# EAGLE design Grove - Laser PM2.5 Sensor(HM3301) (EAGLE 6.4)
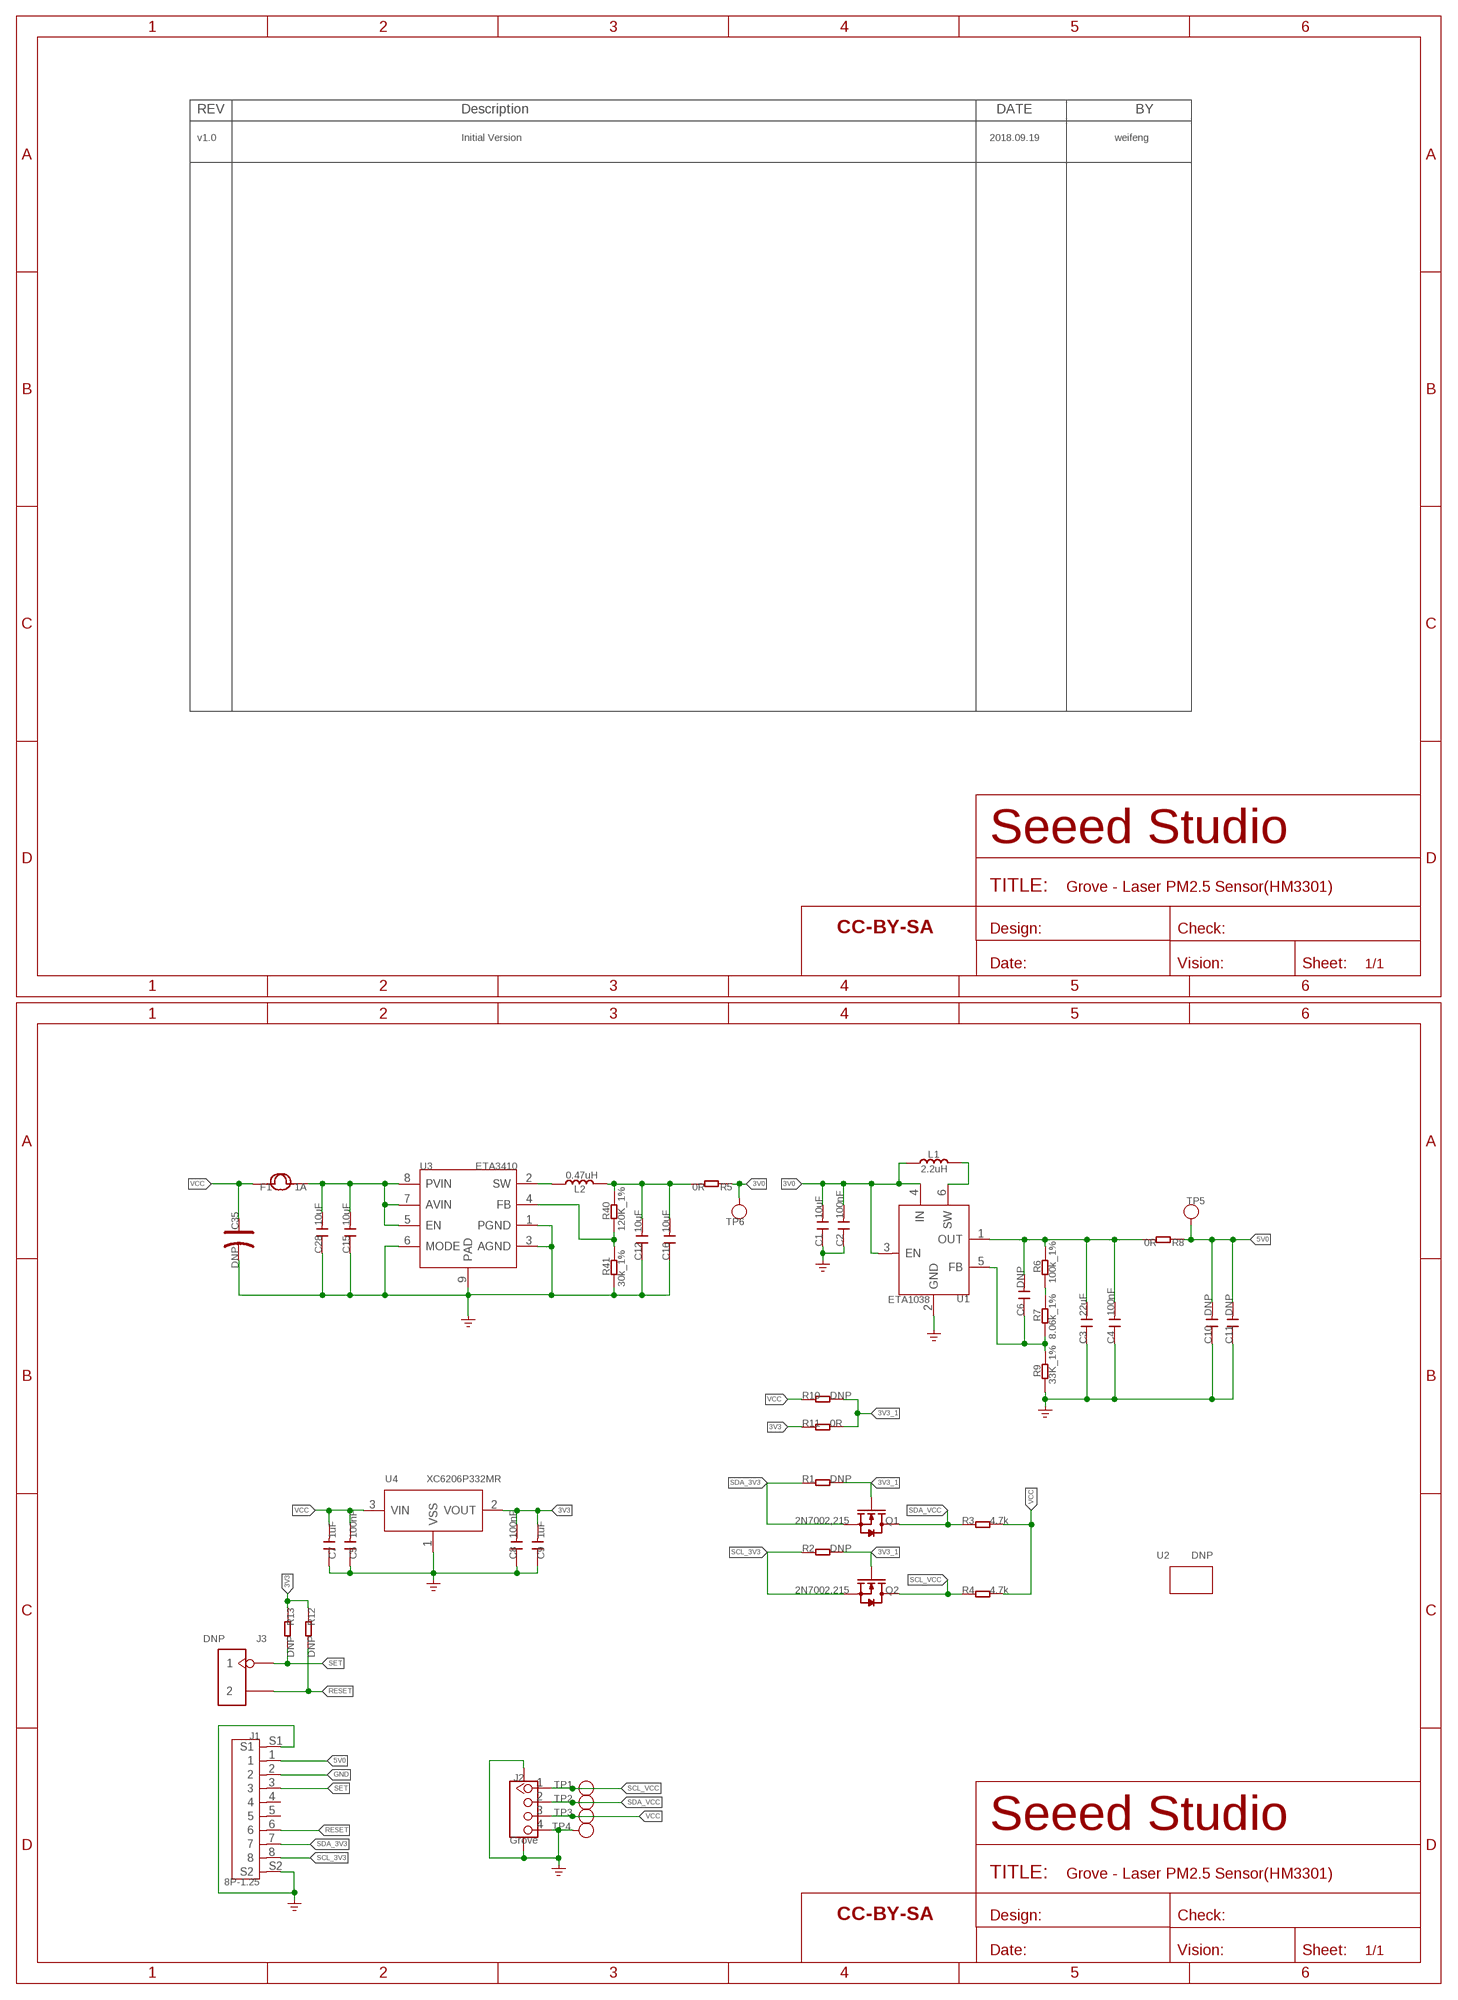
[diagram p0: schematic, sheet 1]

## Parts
C1  10uF  C-0603  [C0603]
C2  100nF  C-0603  [C0603]
C3  22uF  C-0805  [C0805]
C4  100nF  C-0603  [C0603]
C5  100nF  C-0603  [C0603]
C6  DNP  C-0603  [C0603]
C7  1uF  C-0603  [C0603]
C8  100nF  C-0603  [C0603]
C9  1uF  C-0603  [C0603]
C10  DNP  C-0805  [C0805]
C11  DNP  C-0603  [C0603]
C12  10uF  C-0603  [C0603]
C15  10uF  C-0603  [C0603]
C16  10uF  C-0603  [C0603]
C28  10uF  C-0603  [C0603]
C35  DNP  CAP-POLAR-AVX-B  [AVX-B]
F1  1A  FUSE-0805  [F0805]
FR1  SEEEDSTUDIO-OPEN-SCH-FRAME  [SEEEDSTUDIO-PCB-FRAME]
J1  8P-1.25  HEADER-8+2P  [HEADER8+2P-SMD-1.25-15X3.5MM]
J2  Grove  GROVE-CONNECTOR-SMD'90D'  [HW4-SMD-2.0-90D]
J3  DNP  HEADER-2P-65/35MIL  [H2-2.54]
L1  2.2uH  INDUCTOR/FERRITE-BEAD'0806'  [L0806]
L2  0.47uH  L-MPM201610SR33_T  [L201610]
Q1  2N7002,215  MOSFET-N'SOT23'  [SOT-23]
Q2  2N7002,215  MOSFET-N'SOT23'  [SOT-23]
R1  DNP  R-0603  [R0603]
R2  DNP  R-0603  [R0603]
R3  4.7k  R-0603  [R0603]
R4  4.7k  R-0603  [R0603]
R5  0R  R-0603  [R0603]
R6  100k_1%  R-0603  [R0603]
R7  8.06k_1%  R-0603  [R0603]
R8  0R  R-0603  [R0603]
R9  33K_1%  R-0603  [R0603]
R10  DNP  R-0603  [R0603]
R11  0R  R-0603  [R0603]
R12  DNP  R-0603  [R0603]
R13  DNP  R-0603  [R0603]
R40  120K_1%  R-0603  [R0603]
R41  30k_1%  R-0603  [R0603]
TP1  TEST-POINT'4545'  [TP-D45MIL]
TP2  TEST-POINT'4545'  [TP-D45MIL]
TP3  TEST-POINT'4545'  [TP-D45MIL]
TP4  TEST-POINT'4545'  [TP-D45MIL]
TP5  TEST-POINT'4545'  [TP-D45MIL]
TP6  TEST-POINT'4545'  [TP-D45MIL]
U1  ETA1038  CONVERTER-ETA1038  [SOT-23-6]
U2  DNP  GROVE-80X40MM  [GROVE-80X40MM]
U3  ETA3410  CONVERTER-ETA3410  [DFN8G-0.5-2X2MM]
U4  XC6206P332MR  PMIC-XC6206PMR  [SOT-23]
U$4  SEEEDSTUDIO-OPEN-SCH-FRAME  [SEEEDSTUDIO-PCB-FRAME]

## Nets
3V0: C1.2 C2.2 L1.1 R5.1 TP6.T U1.3(EN) U1.4(IN)
3V3: C8.2 C9.2 R11.1 R12.1 R13.1 U4.2(VOUT)
3V3_1: Q1.1(G) Q2.1(G) R1.2 R2.2 R10.2 R11.2
5V0: C10.2 C11.2 J1.1 R8.1 TP5.T
GND: C1.1 C2.1 C3.1 C4.1 C5.1 C7.1 C8.1 C9.1 C10.1 C11.1 C12.1 C15.1 C16.1 C28.1 C35.- J1.2 J1.S1 J1.S2 J2.4 J2.SS1 J2.SS2 R9.2 R41.1 TP4.T U1.2(GND) U3.1(PGND) U3.3(AGND) U3.6(MODE) U3.9(PAD) U4.1(VSS) ; supply symbol labelled GND_POWER
N$7: C15.2 C28.2 F1.2 U3.5(EN) U3.7(AVIN) U3.8(PVIN)
N$8: L1.2 U1.6(SW)
N$9: C3.2 C4.2 C6.2 R6.1 R8.2 U1.1(OUT)
N$10: R6.2 R7.1
N$11: C6.1 R7.2 R9.1 U1.5(FB)
N$21: R40.1 R41.2 U3.4(FB)
N$29: L2.1 U3.2(SW)
N$64: C12.2 C16.2 L2.2 R5.2 R40.2
RESET: J1.6 J3.2 R12.2
SCL_3V3: J1.8 Q2.2(S) R2.1
SCL_VCC: J2.1 Q2.3(D) R4.1 TP1.T
SDA_3V3: J1.7 Q1.2(S) R1.1
SDA_VCC: J2.2 Q1.3(D) R3.1 TP2.T
SET: J1.3 J3.1 R13.2
VCC: C5.2 C7.2 C35.+ F1.1 J2.3 R3.2 R4.2 R10.1 TP3.T U4.3(VIN)
Unconnected: J1.4 J1.5

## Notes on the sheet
- v1.0 | Initial Version | 2018.09.19 | weifeng
- Vout=(R3+R4+R9)/R9x1.17V

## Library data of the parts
C1-C12 C15 C16 C28 = Discrete-small:C*: Ceramic Capacitors
C35 = Discrete-new:CAP-POLAR: Electrolytic Capacitors,Tantalum Capacitors and Super Capacitors
F1 = Discrete-new:FUSE
FR1 U$4 = moudle-new:SEEEDSTUDIO-OPEN-SCH-FRAME
J1 = Connector-new:HEADER-8+2P
J2 = Connector-new:GROVE-CONNECTOR-SMD: 4P-SMD-2.0:320110030;4P-SMD-2.0-90D:320110032
J3 = Connector-new:HEADER-2P
L1 = Discrete-new:INDUCTOR/FERRITE-BEAD
L2 = Discrete-new:L
Q1 Q2 = Discrete-new:MOSFET-N
R1-R13 R40 R41 = Discrete-small:R*
TP1-TP6 = Discrete-new:TEST-POINT; PARTNO: DNP
U1 = IC-new:CONVERTER-ETA1038
U2 = moudle-new:GROVE
U3 = IC-new:CONVERTER-ETA3410: 3MHZ 2A High Step-Down Converter in DFN2x2-8L Package
U4 = IC-new:PMIC-XC6206P: LOW ESR Cap.Compatible Positive Voltage Regulators

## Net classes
3 usbvcc: width 0.203 mm, drill 0.305 mm, clearance 0.203 mm

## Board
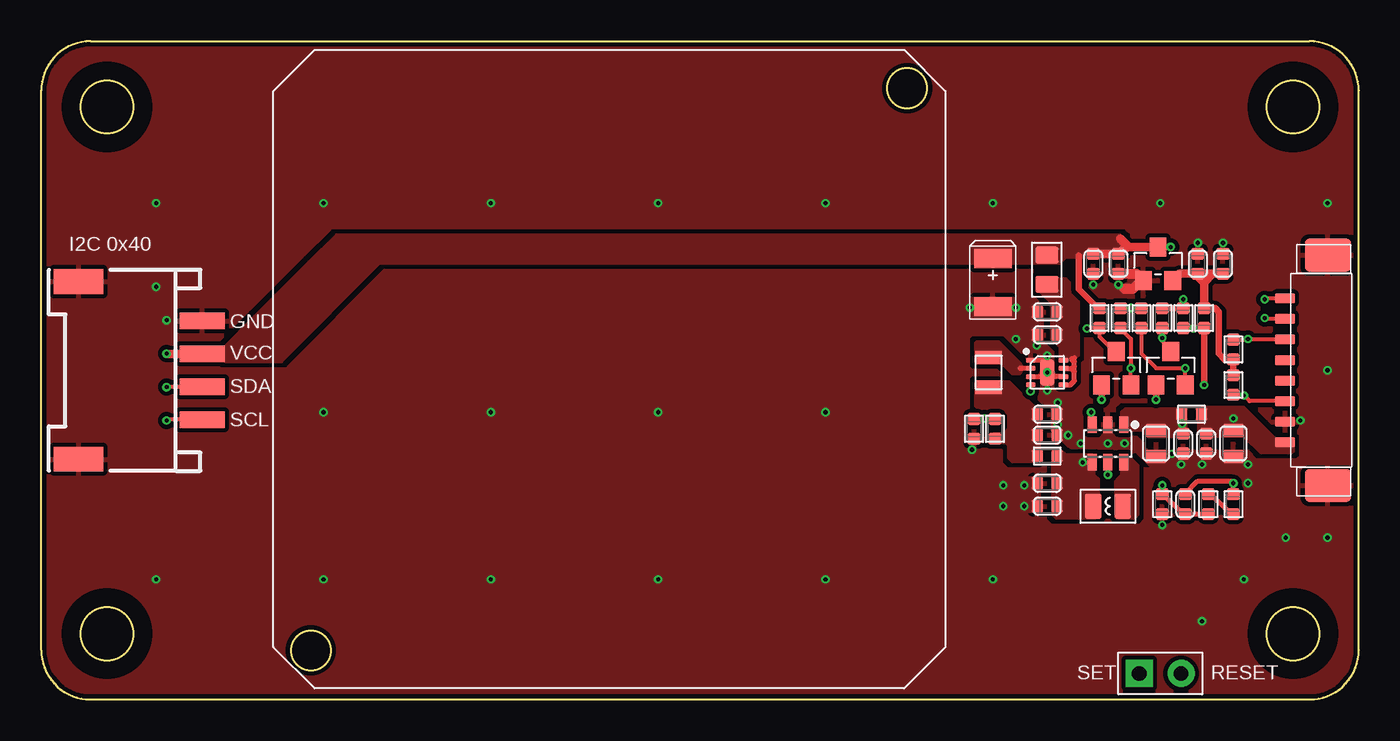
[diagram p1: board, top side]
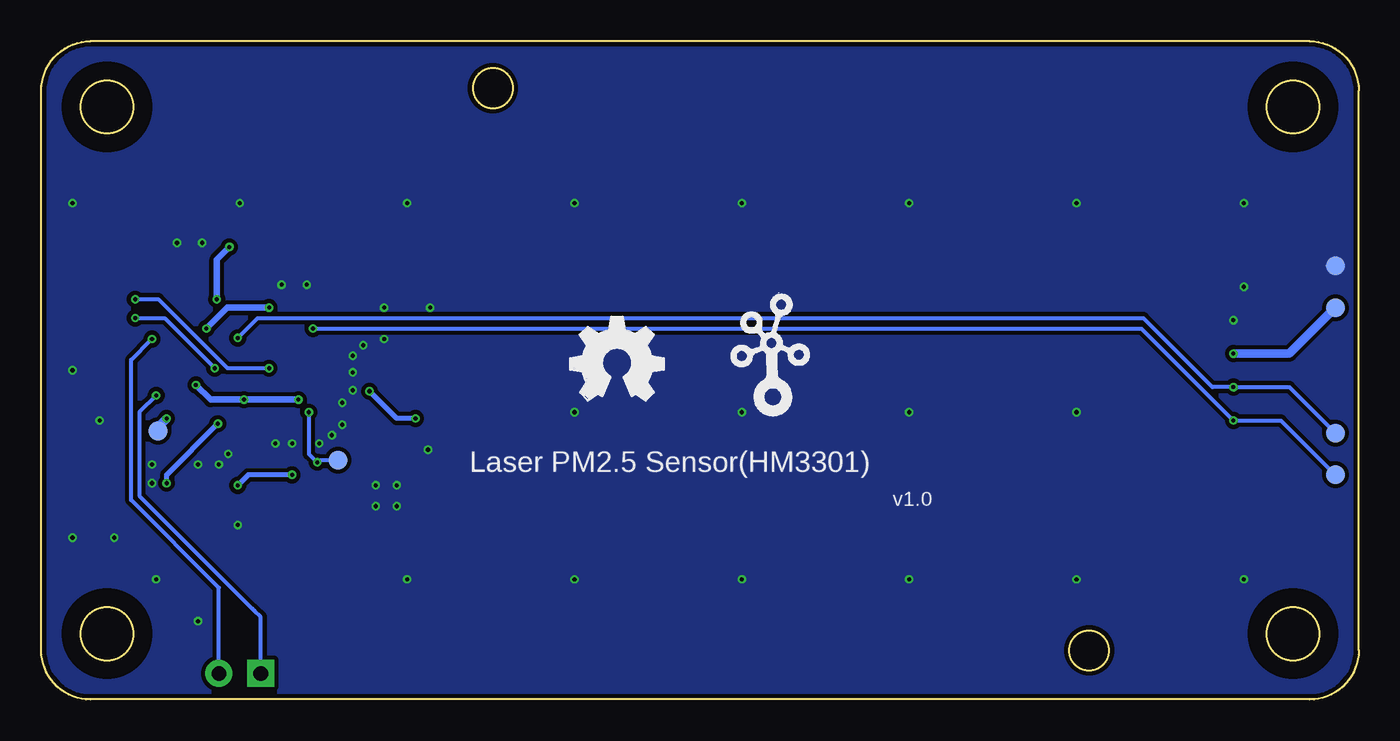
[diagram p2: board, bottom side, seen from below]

Size 80 x 40 mm. Coordinates in mm from the lower left corner, seen from the top.
Outline: circle at 16.38,2.98 radius 1.2
Outline: circle at 52.57,37.14 radius 1.2
Copper layers (1*16): Top 0.035mm / dielectric 1.5mm / Bottom 0.035mm
Design rules "SeeedStudio_2layer_DRU_no_angle_20140221 *": minimum track width 1mil, minimum drill 10mil, track to track 6mil, track to pad 6mil, pad to pad 6mil, via to via 6mil, smd to smd 0mil, copper to edge 10mil, drill to drill 10mil, minimum pad ring 4mil, minimum via ring 4mil, stop-mask expansion 2mil, vias tented up to drill 25mil, thermal gap 10mil

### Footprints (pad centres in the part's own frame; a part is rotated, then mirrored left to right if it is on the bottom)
C0603 = smd 0.762 x 0.696: 1 0,0.602; 2 0,-0.602
C0805 = smd 0.819 x 1.27: 1 -0.79,0; 2 0.79,0
AVX-B = smd 1.143 x 2.286: + 1.46,0; - -1.46,0
F0805 = smd 1.016 x 1.397: 1 -0.889,0; 2 0.889,0
HEADER8+2P-SMD-1.25-15X3.5MM = smd 0.6 x 1.2: 1 -4.375,2.2; 2 -3.125,2.2; 3 -1.875,2.2; 4 -0.625,2.2; 5 0.625,2.2; 6 1.875,2.2; 7 3.125,2.2; 8 4.375,2.2 | smd 2 x 2.8: S1 -7,-0.4; S2 7,-0.4
HW4-SMD-2.0-90D = smd 1.01 x 2.74: 1 -3,-0.1; 2 -1,-0.1; 3 1,-0.1; 4 3,-0.1 | smd 1.5 x 3: SS1 -5.4,7.4; SS2 5.4,7.4
H2-2.54 = drill 0.889 pad 1.651 square: 1 0,1.27 | drill 0.889 pad 1.651: 2 0,-1.27
L0806 = smd 1.016 x 1.524: 1 -0.889,0; 2 0.889,0
L201610 = smd 0.8 x 1.6: 1 -0.9,0; 2 0.9,0
SOT-23 = smd 1.143 x 1.016: 1 1.016,-0.889; 2 1.016,0.889; 3 -1.016,0
R0603 = smd 0.762 x 0.696: 1 0,0.602; 2 0,-0.602
TP-D45MIL = smd 1.143 x 1.143: T 0,0
SOT-23-6 = smd 0.55 x 1.016: 1 -0.95,-1.143; 2 0,-1.143; 3 0.95,-1.143; 4 0.95,1.143; 5 0,1.143; 6 -0.95,1.143
DFN8G-0.5-2X2MM = smd 0.6 x 0.3: 1 -1,0.75; 2 -1,0.25; 3 -1,-0.25; 4 -1,-0.75; 5 1,-0.75; 6 1,-0.25; 7 1,0.25; 8 1,0.75 | smd 0.9 x 1.6: 9 0,0
SOT-23' = smd 1.016 x 1.143: 1 -0.889,-1.016; 2 0.889,-1.016; 3 0,1.016

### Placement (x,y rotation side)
C1  61.08,11.74 90 top
C2  61.08,13.14 90 top
C3  67.69,15.55 90 top
C4  69.34,15.55 180 top
C5  65.4,26.48 180 top
C6  69.46,11.87 180 top
C7  63.88,26.48 180 top
C8  71.75,26.48 0 top
C9  70.23,26.48 0 top
C10  72.38,15.55 90 top
C11  70.73,15.55 180 top
C12  61.08,17.33 270 top
C15  61.08,22.16 90 top
C16  61.08,16.06 270 top
C28  61.08,23.56 90 top
C35  57.78,25.33 90 top
F1  61.06,26.12 270 top
FR1  not placed on the board
J1  77.72,20 90 top
J2  9.67,20 90 top
J3  67.94,1.59 90 top
L1  64.77,11.74 0 top
L2  57.53,19.87 270 top
Q1  68.58,20.13 270 top
Q2  65.27,20.13 270 top
R1  66.8,23.18 180 top
R2  65.53,23.18 180 top
R3  68.07,23.18 180 top
R4  64.26,23.18 180 top
R5  61.08,14.79 270 top
R6  72.38,11.87 0 top
R7  70.86,11.87 0 top
R8  69.84,17.33 270 top
R9  68.07,11.87 0 top
R10  69.34,23.18 0 top
R11  70.61,23.18 0 top
R12  72.38,21.27 180 top
R13  72.38,19.11 0 top
R40  57.91,16.44 0 top
R41  56.64,16.44 180 top
TP1  1.43,13.65 0 bottom
TP2  1.43,16.19 0 bottom
TP3  1.43,23.81 0 bottom
TP4  1.43,26.35 0 bottom
TP5  72.89,16.32 270 bottom
TP6  61.97,14.54 180 bottom
U1  64.77,15.55 180 top
U2  40,20 0 top
U3  61.08,19.87 0 top
U4  XC6206P332MR  [SOT-23']  67.81,26.48 0 top
U$4  not placed on the board
U$5  [OSHW_FILLX200_NOTEXT]  47.88,18.16 0 bottom
U$7  [TWIGLOGO]  35.63,18.18 0 bottom

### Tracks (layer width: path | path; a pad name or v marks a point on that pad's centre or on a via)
3V0  (via drill 0.25 pad 0.51)
  Top 0.254: U1.3 63.81,17.39 v63.75,17.46 | v63.24,14.41 U1.4
  Bottom 0.254: v63.75,17.46 63.75,14.92 v63.24,14.41 63.11,14.54 TP6.T
  pour Top (isolate 0.254, no thermals): 63.62,14.92 62.23,14.92 61.97,15.17 61.46,15.17 61.34,15.05 61.34,11.24 61.59,10.98 64,10.98 64.26,11.24 64.26,13.4 64,13.65 64,14.79 63.88,14.92
3V3
  Top 0.406: R11.1 71.28,23.78 71.5,23.56 71.5,21.02 71.84,20.67 R12.1 R13.1
  Top 0.508: 70.61,25.88 C9.2 69.12,25.88 U4.2 | 70.61,25.88 C8.2 | R11.1 70.61,25.33 | 70.61,25.33 70.61,25.88 | 70.61,25.33 70.1,25.84 | 70.61,25.33 71.11,25.84
3V3_1  (via drill 0.25 pad 0.51)
  Top 0.406: v70.61,19.11 R11.2 70,22.57 v69.97,22.54 69.94,22.57 R10.2 | v67.69,18.22 Q1.1 | v64.38,18.22 Q2.1 | R2.2 65.56,23.81 v66.16,23.81 66.19,23.78 R1.2
  Bottom 0.406: v64.38,18.22 v67.69,18.22 69.72,18.22 v70.61,19.11 | v69.97,22.54 68.7,23.81 v66.16,23.81
5V0  (via drill 0.25 pad 0.51)
  Bottom 0.508: TP5.T 72.89,16.57 v72.38,17.08
  pour Top (isolate 0.254, no thermals): 75.56,14.92 74.04,14.92 73.02,15.94 70.48,15.94 70.23,16.19 70.23,17.59 70.48,17.84 73.02,17.84 74.92,15.94 75.94,15.94 76.07,15.81 76.07,15.05 75.94,14.92
GND  (via drill 0.25 pad 0.51)
  Top 0.305: U3.3 60.83,19.62 U3.9 61.33,19.62 U3.6 | U3.1 60.94,20.62 60.95,20.64
  Top 0.61: 65.78,24.95 66.29,24.95 66.8,25.46 U4.1 66.51,25.88 C5.1
  other vias: 56.38,23.81 59.18,23.81 59.18,21.91 61.08,19.87 61.08,20.89 61.08,18.79 60.45,21.52 61.72,18.03 61.72,16.7 62.35,16.06 64.77,15.55 65.78,15.55 63.11,15.55 68.64,14.92 69.21,14.29 70.48,14.29 73.27,14.29 73.27,13.14 68.07,10.6 63.88,25.21 65.4,25.21 70.23,27.75 71.75,27.75 59.69,11.74 59.69,13.02 58.41,13.02 58.41,11.74 56.51,15.17 76.45,16.95 7.62,23.05 6.98,25.08 6.98,30.16 17.14,30.16 27.3,30.16 37.46,30.16 47.62,30.16 57.78,30.16 67.94,30.16 78.1,30.16 78.1,20 78.1,9.84 75.56,9.84 73.02,7.3 70.48,4.76 57.78,7.3 47.62,7.3 37.46,7.3 6.98,7.3 27.3,7.3 17.14,7.3 17.14,17.46 27.3,17.46 37.46,17.46 47.62,17.46
  pour Top (isolate 0.254, no thermals): 73.4,13.78 67.69,13.78 66.16,15.3 62.35,15.3 61.34,16.32 61.34,18.09 60.7,18.73 60.7,20.89 60.07,21.52 59.18,21.52 58.41,22.29 56.51,22.29 56.13,22.67 56.13,24.19 56.38,24.45 60.19,24.45 60.83,23.81 60.83,21.78 61.46,21.14 61.46,18.98 63.24,17.21 63.24,16.19 63.5,15.94 64.26,15.94 64.51,16.19 64.51,16.95 64.64,17.08 64.89,17.08 65.02,16.95 65.02,16.19 65.27,15.94 66.42,15.94 67.18,15.17 73.27,15.17 73.53,14.92 73.53,13.9
  pour Top (isolate 0.254, no thermals): 60.45,13.52 58.03,13.52 57.78,13.27 57.78,11.62 58.03,11.36 60.45,11.36 60.7,11.62 60.7,13.4 60.57,13.52
  pour Bottom (isolate 0.254, rank 6): -0.64,40.32 80.64,40.32 80.64,-0.32 -0.64,-0.32
  pour Top (isolate 0.254, rank 6): -0.64,40.32 80.64,40.32 80.64,-0.32 -0.64,-0.32
N$7
  Top 0.305: U3.7 62.34,20.12 62.55,20.12 | 62.55,20.12 62.6,20.12 62.73,20.25 | 62.73,20.25 62.73,20.51 | 62.73,20.51 62.73,20.76 | 62.73,20.51 62.54,20.7 | U3.5 62.49,19.12 62.73,19.36 62.73,19.94 | 62.73,19.94 62.73,20.25 | 62.55,20.12 62.73,19.94
  pour Top (isolate 0.254, no thermals): 60.95,25.59 60.57,25.59 60.45,25.46 60.45,24.95 61.34,24.06 61.34,21.91 61.84,21.4 61.84,20.76 61.97,20.64 62.73,20.64 62.99,20.89 62.99,24.19 62.48,24.7 62.48,25.33 62.23,25.59
N$8
  pour Top (isolate 0.254, no thermals): 65.91,14.67 65.65,14.67 65.53,14.54 65.53,13.65 65.15,13.27 65.15,11.24 65.4,10.98 66.42,10.98 66.67,11.24 66.67,14.21 66.21,14.67
N$9  (via drill 0.25 pad 0.51)
  Top 0.305: R6.1 v72.38,13.14 72.26,13.27 70.23,13.27 69.46,12.51 C6.2 | C4.2 69.34,16.7 v69.27,16.76 69.24,16.79 R8.2
  Bottom 0.305: v72.38,13.14 72.38,13.65 v69.27,16.76
  pour Top (isolate 0.254, no thermals): 69.46,17.71 65.78,17.71 65.53,17.46 65.53,16.5 65.71,16.32 66.8,16.32 67.18,15.94 69.46,15.94 69.59,16.06 69.59,17.59
N$10
  Top 0.305: R6.2 72.22,11.27 71.02,12.47 R7.1
N$11  (via drill 0.25 pad 0.51)
  Top 0.305: U1.5 v64.77,13.65 | v68.07,13.02 R9.1 68.1,12.47 69.3,11.27 C6.1 R7.2
  Bottom 0.305: v64.77,13.65 67.43,13.65 v68.07,13.02
N$21  (via drill 0.25 pad 0.51)
  Top 0.305: U3.4 60.08,18.75 v60.07,18.73 | R40.1 57.3,17.05 v57.27,17.08 57.24,17.05 R41.2
  Bottom 0.305: v57.27,17.08 58.41,17.08 v60.07,18.73
N$29
  Top 0.305: U3.2 59.44,20.12 59.43,20.13
  pour Top (isolate 0.254, no thermals): 60.13,20.25 59.69,20.25 58.16,21.78 56.76,21.78 56.64,21.65 56.64,20.51 56.76,20.38 58.29,20.38 58.92,19.75 59.43,19.75 59.69,20 60.13,20 60.19,20.06 60.19,20.19
N$64
  pour Top (isolate 0.254, no thermals): 57.65,19.36 56.76,19.36 56.64,19.24 56.64,17.84 56.89,17.59 58.41,17.59 58.67,17.33 58.67,16.44 58.41,16.19 57.78,16.19 57.65,16.06 57.65,15.68 57.78,15.55 58.54,15.55 58.67,15.43 58.67,14.67 58.92,14.41 60.45,14.41 60.7,14.67 60.7,17.46 59.43,18.73 58.8,19.36
RESET  (via drill 0.25 pad 0.51)
  Top 0.254: R12.2 73.24,21.87 v73.27,21.91 73.3,21.88 J1.6
  Bottom 0.254: J3.2 69.21,6.79 74.54,12.13 74.54,20.64 v73.27,21.91
SCL_3V3  (via drill 0.25 pad 0.51)
  Top 0.254: Q2.2 v66.16,20.13 66.16,21.91 65.53,22.54 R2.1 | J1.8 74.35,24.38 v74.29,24.32
  Bottom 0.254: v66.16,20.13 68.7,20.13 72.89,24.32 v74.29,24.32
SCL_VCC  (via drill 0.25 pad 0.51)
  Top 0.254: J2.1 7.66,17 v7.62,16.95 | Q2.3 65.15,21.14 64.26,22.03 R4.1 63.53,22.57 v63.5,22.54
  Bottom 0.254: TP1.T 4.73,16.95 v7.62,16.95 13.2,22.54 v63.5,22.54
SDA_3V3  (via drill 0.25 pad 0.51)
  Top 0.254: R1.1 66.8,21.02 67.69,20.13 v69.46,20.13 Q1.2 | J1.7 74.34,23.12 v74.29,23.18
  Bottom 0.254: v69.46,20.13 72.51,23.18 v74.29,23.18
SDA_VCC  (via drill 0.25 pad 0.51)
  Top 0.254: J2.2 7.63,19 v7.62,18.98 | R3.1 v68.07,21.97 68.07,21.78 68.58,21.27 Q1.3
  Bottom 0.254: TP2.T 4.22,18.98 v7.62,18.98 8.89,18.98 13.08,23.18 66.86,23.18 v68.07,21.97
SET  (via drill 0.25 pad 0.51)
  Top 0.254: R13.2 72.99,18.51 v73.02,18.48 73.37,18.12 J1.3
  Bottom 0.254: v73.02,18.48 74.04,17.46 74.04,12.38 67.18,5.52 67.05,5.39 66.67,5.01 J3.1
VCC  (via drill 0.25 pad 0.51)
  Top 0.406: R3.2 R10.1 v69.34,24.32 | v68.58,27.49 U4.3 | R4.2 64.16,23.78 62.99,24.95 62.99,26.98
  Top 0.508: J2.3 7.63,21 v7.62,21.02 | U4.3 66.54,27.49 66.03,27.49 | 66.03,27.49 65.81,27.49 C5.2 C7.2 | 66.03,27.49 65.53,28 | 66.29,27.49 65.91,27.49 65.4,26.98
  Bottom 0.406: v69.34,24.32 69.34,26.73 v68.58,27.49
  Bottom 0.508: v7.62,21.02 4.22,21.02 TP3.T
  pour Top (isolate 0.254, no thermals): 65.53,26.86 62.23,26.86 61.84,26.48 20.57,26.48 14.6,20.51 11.17,20.51 11.04,20.64 11.04,21.4 12.95,23.3 16.25,26.6 17.9,28.26 65.53,28.26 65.78,28 65.78,27.11

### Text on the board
tPlace: I2C 0x40 | GND | VCC | SDA | SCL | SET | RESET
bPlace: Laser PM2.5 Sensor(HM3301) | v1.0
